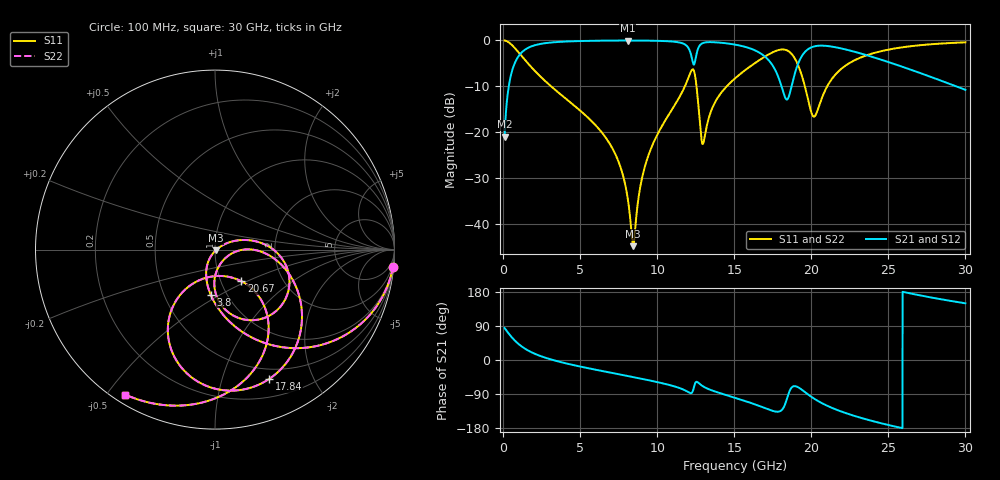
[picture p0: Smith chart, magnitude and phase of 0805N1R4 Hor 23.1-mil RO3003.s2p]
# GHz S MA R 50
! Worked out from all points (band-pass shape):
!   3201 points, 100 MHz to 30 GHz, reference 50 ohm
!   highest |S21| = -0.05 dB at 8.089 GHz (marker M1); lowest = -21.0 dB at 100 MHz (marker M2)
!   |S21| within 3 dB of the highest: 1.097 GHz to 12.19 GHz (11.09 GHz wide, 167 % of centre); 12.55 GHz to 16.8 GHz (4.251 GHz wide, 29 % of centre)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
!   lowest |S11| = -44.8 dB at 8.444 GHz (marker M3), VSWR 1.01, Z = 50.4 - j0.416 ohm
!   |S11| at or under -10 dB: 3.108 GHz to 11.8 GHz (8.693 GHz wide, 117 % of centre); 12.55 GHz to 14.52 GHz (1.969 GHz wide, 14.5 % of centre); 19.58 GHz to 21.04 GHz (1.455 GHz wide, 7.16 % of centre)
!   |S22| runs from -44.8 to 0.0 dB; largest |S21 - S12| = 0
!   S11 on the Smith chart (normalised r, x): 100 MHz: 1, -20; 3.8 GHz: 0.84, -0.45; 17.84 GHz: 0.39, -1.43; 20.67 GHz: 1.25, -0.46; 30 GHz: 0.03, -0.56
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0.1  0.996 -5.7  0.08945 84.3  0.08945 84.3  0.996 -5.7
0.4644063  0.9226 -25.2  0.3853 64.8  0.3853 64.8  0.9226 -25.2
0.997  0.7425 -47.4  0.6688 42.5  0.6688 42.5  0.7425 -47.4
3.800125  0.2523 -95.4  0.9646 -6.1  0.9646 -6.1  0.2523 -95.4
5.089563  0.1667 -106.8  0.9823 -18.0  0.9823 -18.0  0.1667 -106.8
7.1265  0.06507 -120.5  0.993 -34.6  0.993 -34.6  0.06507 -120.5
8.088906  0.01901 -115.7  0.9941 -42.2  0.9941 -42.2  0.01901 -115.7
8.443969  0.005734 -46.0  0.994 -45.1  0.994 -45.1  0.005734 -46.0
9.088688  0.03566 29.1  0.9926 -50.4  0.9926 -50.4  0.03566 29.1
10.06978  0.09822 26.1  0.9863 -58.9  0.9863 -58.9  0.09822 26.1
11.71428  0.2942 4.0  0.9168 -78.3  0.9168 -78.3  0.2942 4.0
12.28425  0.4825 -38.1  0.6042 -84.6  0.6042 -84.6  0.4825 -38.1
12.62063  0.244 -89.1  0.7818 -58.5  0.7818 -58.5  0.244 -89.1
12.99437  0.07594 -34.5  0.9368 -70.0  0.9368 -70.0  0.07594 -34.5
15.05  0.3846 -13.4  0.8975 -99.6  0.8975 -99.6  0.3846 -13.4
17.84378  0.7811 -67.2  0.4054 -136.5  0.4054 -136.5  0.7811 -67.2
18.43244  0.776 -89.6  0.2264 -100.4  0.2264 -100.4  0.776 -89.6
19.03978  0.5857 -115.5  0.4979 -69.9  0.4979 -69.9  0.5857 -115.5
20.03956  0.1577 -103.3  0.8422 -98.1  0.8422 -98.1  0.1577 -103.3
20.66559  0.2295 -50.2  0.8748 -113.4  0.8748 -113.4  0.2295 -50.2
25.01978  0.7924 -84.0  0.5784 -171.7  0.5784 -171.7  0.7924 -84.0
30  0.95 -121.7  0.2887 149.6  0.2887 149.6  0.95 -121.7
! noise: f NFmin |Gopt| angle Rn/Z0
0.1  0.001106  0.9485  1.537  0.004814
3.417  0.007435  0.7433  19.42  0.00565
6.743  0.01302  0.7197  36.6  0.008316
10.06  0.02168  0.751  52.99  0.01413
13.39  0.04942  0.8508  69.18  0.04798
16.7  0.08733  0.8952  84.17  0.1005
20.03  0.1362  0.9201  98.9  0.1597
23.35  0.08086  0.8521  111.9  0.03705
26.67  0.08598  0.8464  124.2  0.02666
30  0.1064  0.8648  136.4  0.02409
